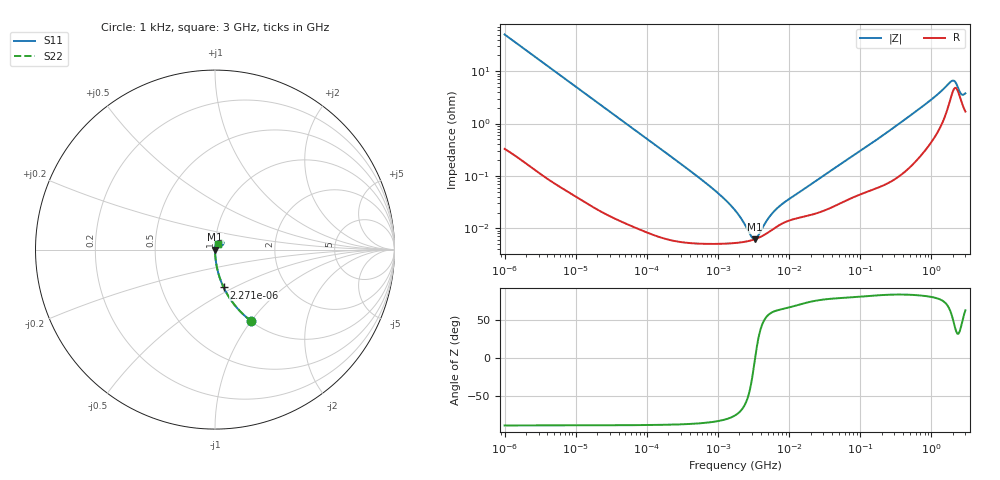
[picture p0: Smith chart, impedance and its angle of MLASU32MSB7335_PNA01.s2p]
! MLASU32MSB7335_PNA01  S-PARAMETER MODEL  ( Standard Model )
! Model Generated by TAIYO YUDEN Corporation (http://www.ty-top.com)
! Version 1.0
! TAIYO YUDEN Control No. 220601
! Copyright(c) 2017 TAIYO YUDEN CO.,LTD. All Rights Reserved.
! Product Description (link to TY-COMPAS)
! https://ds.yuden.co.jp/TYCOMPAS/or/detail?pn=MLASU32MSB7335KPNA01&u=M
! Products Name : Multilayer Ceramic Capacitors
! Characteristics :
!  Capacitance : 3.3 [uF] , Rated Voltage : 50 [V] , TCC : X7R
!  Case Size : 3.2 x 2.5 / 0.126 x 0.098 [mm/inch] , Thickness : 2.5 / 0.098 [mm/inch]
!  (Conditions: Temperature = 25 [degC] , DC Bias Voltage = 0 [V])
! External Node Assignments :
!  1  o---| |---o  2
! GND o---------o GND
! Frequency Range : 1kHz  -  3GHz  [ 401 STEP ]
# MHZ S RI R 50
! Freq[MHz].  S11 Real  S11 Imag  S21 Real  S21 Imag  S12 Real  S12 Imag  S22 Real  S22 Imag
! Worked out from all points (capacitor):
!   401 points, 1 kHz to 3 GHz, reference 50 ohm
!   read as one part in series: C = 3.17 uF near 1.077 kHz
!   lowest |Z| = 6.2 mohm at 3.265 MHz (marker M1)
!   series resonance near 3.324 MHz, so ESL is about 720 pH
!   S11 on the Smith chart (normalised r, x): 1 kHz: 1.01, -1.00; 2.271 kHz: 1.00, -0.44; 3 GHz: 1.03, +0.07
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0.001  0.2023 -0.3985  0.7977 0.3985  0.7977 0.3985  0.2023 -0.3985
0.001507  0.1016 -0.2987  0.8984 0.2987  0.8984 0.2987  0.1016 -0.2987
0.002271  0.0481 -0.2106  0.9519 0.2106  0.9519 0.2106  0.0481 -0.2106
0.004787  0.0117 -0.1041  0.9883 0.1041  0.9883 0.1041  0.0117 -0.1041
0.01216  0.00207 -0.0416  0.9979 0.0416  0.9979 0.0416  0.00207 -0.0416
0.147855  8.07e-05 -0.00346  0.9999 0.00346  0.9999 0.00346  8.07e-05 -0.00346
0.791611  5.09e-05 -0.000613  0.9999 0.000613  0.9999 0.000613  5.09e-05 -0.000613
1.238299  5.12e-05 -0.000358  0.9999 0.000358  0.9999 0.000358  5.12e-05 -0.000358
1.732051  5.26e-05 -0.000216  0.9999 0.000216  0.9999 0.000216  5.26e-05 -0.000216
2.514714  5.63e-05 -8.73e-05  0.9999 8.73e-05  0.9999 8.73e-05  5.63e-05 -8.73e-05
2.709407  5.75e-05 -6.35e-05  0.9999 6.35e-05  0.9999 6.35e-05  5.75e-05 -6.35e-05
3.264662  6.18e-05 -5.48e-06  0.9999 5.48e-06  0.9999 5.48e-06  6.18e-05 -5.48e-06
4.083148  7.03e-05 6.32e-05  0.9999 -6.32e-05  0.9999 -6.32e-05  7.03e-05 6.32e-05
5.711239  9.34e-05 0.000165  0.9999 -0.000165  0.9999 -0.000165  9.34e-05 0.000165
7.143107  0.000114 0.000232  0.9999 -0.000232  0.9999 -0.000232  0.000114 0.000232
21.06097  0.000184 0.000695  0.9998 -0.000695  0.9998 -0.000695  0.000184 0.000695
256.0921  0.000805 0.00725  0.9992 -0.00725  0.9992 -0.00725  0.000805 0.00725
944.3747  0.00468 0.0266  0.9953 -0.0266  0.9953 -0.0266  0.00468 0.0266
1917.819  0.0361 0.051  0.9639 -0.051  0.9639 -0.051  0.0361 0.051
2144.796  0.0474 0.0373  0.9526 -0.0373  0.9526 -0.0373  0.0474 0.0373
2584.342  0.0282 0.0228  0.9718 -0.0228  0.9718 -0.0228  0.0282 0.0228
3000  0.0178 0.0326  0.9822 -0.0326  0.9822 -0.0326  0.0178 0.0326
